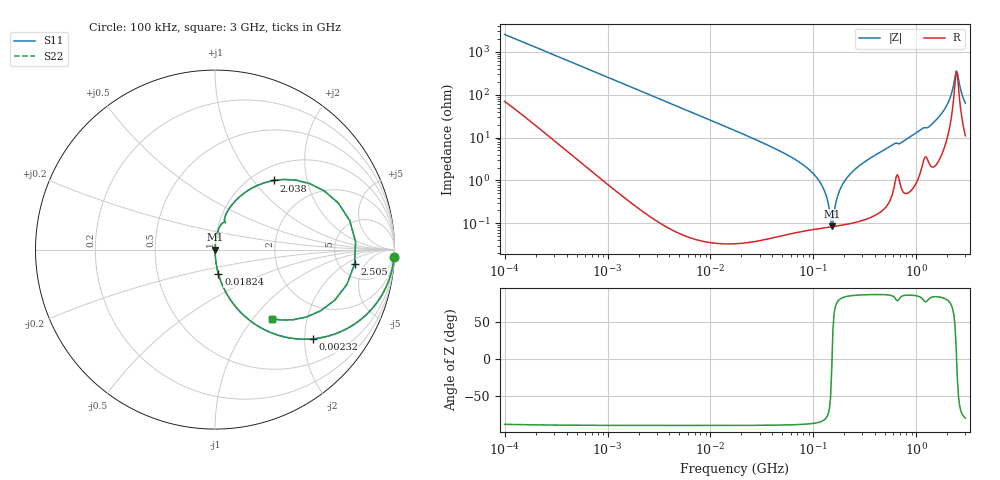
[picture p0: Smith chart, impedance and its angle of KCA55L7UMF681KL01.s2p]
!Murata Part Number: KCA55L7UMF681KL01
!These Parameters are Measured in Series Mode Connection
!Data Generated on Jan 08, 2026
!  o--ll--o
!Port1  Port2
!  o------o
!Operation Temp=25[degC], DC Bias Voltage=0[V]
!Freq. Start=100[kHz] Stop=3[GHz] 401[Steps]
# Hz S RI R 50
!Freq.(Hz) S11(Real) S11(Imag) S21(Real) S21(Imag) S12(Real) S12(Imag) S22(Real) S22(Imag)
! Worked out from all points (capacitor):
!   401 points, 100 kHz to 3 GHz, reference 50 ohm
!   read as one part in series: C = 629 pF near 105.3 kHz
!   lowest |Z| = 84.8 mohm at 150.9 MHz (marker M1)
!   series resonance near 151.7 MHz, so ESL is about 1.7 nH
!   S11 on the Smith chart (normalised r, x): 100 kHz: 2, -50; 2.32 MHz: 1.00, -2.19; 18.24 MHz: 1.00, -0.27; 2.038 GHz: 1.24, +1.28; 2.505 GHz: 6.96, -2.88; 3 GHz: 1.22, -1.25
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100000  0.9973 -0.0395  0.00266 0.0395  0.00266 0.0395  0.9973 -0.0395
562235  0.9524 -0.2101  0.0476 0.2101  0.0476 0.2101  0.9524 -0.2101
1156955  0.8281 -0.3759  0.1719 0.3759  0.1719 0.3759  0.8281 -0.3759
2320182  0.5461 -0.4971  0.4539 0.4971  0.4539 0.4971  0.5461 -0.4971
3161081  0.3934 -0.4878  0.6066 0.4878  0.6066 0.4878  0.3934 -0.4878
6848882  0.1212 -0.3258  0.8788 0.3258  0.8788 0.3258  0.1212 -0.3258
1.77727e7  0.0199 -0.1383  0.9801 0.1383  0.9801 0.1383  0.0199 -0.1383
1.82367e7  0.0189 -0.1348  0.9811 0.1348  0.9811 0.1348  0.0189 -0.1348
5.523785e7  0.00212 -0.0397  0.9979 0.0397  0.9979 0.0397  0.00212 -0.0397
9.738194e7  0.000941 -0.0153  0.9991 0.0153  0.9991 0.0153  0.000941 -0.0153
1.260104e8  0.000817 -0.00622  0.9992 0.00622  0.9992 0.00622  0.000817 -0.00622
1.509232e8  0.00083 -0.000173  0.9992 0.000173  0.9992 0.000173  0.00083 -0.000173
1.589065e8  0.000848 0.00155  0.9992 -0.00155  0.9992 -0.00155  0.000848 0.00155
1.807614e8  0.000923 0.00589  0.9991 -0.00589  0.9991 -0.00589  0.000923 0.00589
2.164987e8  0.00111 0.0122  0.9989 -0.0122  0.9989 -0.0122  0.00111 0.0122
5.475153e8  0.00678 0.0601  0.9932 -0.0601  0.9932 -0.0601  0.00678 0.0601
1.495945e9  0.0684 0.2111  0.9316 -0.2111  0.9316 -0.2111  0.0684 0.2111
2.038117e9  0.326 0.3851  0.674 -0.3851  0.674 -0.3851  0.326 0.3851
2.259438e9  0.6095 0.3265  0.3905 -0.3265  0.3905 -0.3265  0.6095 0.3265
2.504792e9  0.7777 -0.0803  0.2223 0.0803  0.2223 0.0803  0.7777 -0.0803
2.706139e9  0.5877 -0.3417  0.4123 0.3417  0.4123 0.3417  0.5877 -0.3417
3e9  0.3152 -0.3852  0.6848 0.3852  0.6848 0.3852  0.3152 -0.3852
